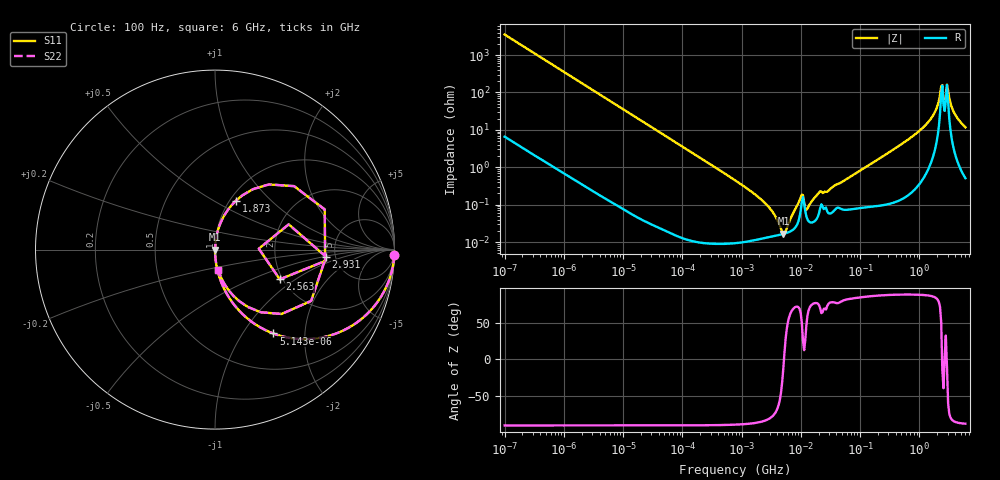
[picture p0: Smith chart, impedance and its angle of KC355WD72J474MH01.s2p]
!Murata Part Number: KC355WD72J474MH01
!These Parameters are Measured in Series Mode Connection
!Data Generated on Mar 13, 2026
!  o--ll--o
!Port1  Port2
!  o------o
!Operation Temp=25[degC], DC Bias Voltage=0[V]
!Freq. Start=100[Hz] Stop=6[GHz] 401[Steps]
# Hz S RI R 50
!Freq.(Hz) S11(Real) S11(Imag) S21(Real) S21(Imag) S12(Real) S12(Imag) S22(Real) S22(Imag)
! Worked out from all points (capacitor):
!   401 points, 100 Hz to 6 GHz, reference 50 ohm
!   read as one part in series: C = 449 nF near 109 Hz
!   lowest |Z| = 16.8 mohm at 5.079 MHz (marker M1)
!   series resonance near 5.199 MHz, so ESL is about 2.1 nH
!   S11 on the Smith chart (normalised r, x): 100 Hz: 1, -71; 5.143 kHz: 1.00, -1.39; 1.873 GHz: 1.07, +0.64; 2.563 GHz: 1.93, -0.76; 2.931 GHz: 4.19, -0.55; 6 GHz: 1.01, -0.23
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100  0.9992 -0.0282  0.000847 0.0282  0.000847 0.0282  0.9992 -0.0282
750  0.957 -0.2019  0.043 0.2019  0.043 0.2019  0.957 -0.2019
2008  0.758 -0.4273  0.242 0.4273  0.242 0.4273  0.758 -0.4273
5143  0.3246 -0.4672  0.6754 0.4672  0.6754 0.4672  0.3246 -0.4672
12041  0.0811 -0.272  0.9189 0.272  0.9189 0.272  0.0811 -0.272
40335  0.00801 -0.0878  0.992 0.0878  0.992 0.0878  0.00801 -0.0878
774597  0.000113 -0.0045  0.9999 0.0045  0.9999 0.0045  0.000113 -0.0045
2713602  0.000133 -0.000948  0.9999 0.000948  0.9999 0.000948  0.000133 -0.000948
5079039  0.000165 -3.23e-05  0.9998 3.23e-05  0.9998 3.23e-05  0.000165 -3.23e-05
9941735  0.000696 0.00138  0.9993 -0.00138  0.9993 -0.00138  0.000696 0.00138
1.300572e7  0.000397 0.0007  0.9996 -0.0007  0.9996 -0.0007  0.000397 0.0007
1.555665e7  0.000336 0.00123  0.9997 -0.00123  0.9997 -0.00123  0.000336 0.00123
2.035112e7  0.000605 0.00205  0.9994 -0.00205  0.9994 -0.00205  0.000605 0.00205
3.124326e8  0.00169 0.0252  0.9983 -0.0252  0.9983 -0.0252  0.00169 0.0252
1.046602e9  0.0136 0.0979  0.9864 -0.0979  0.9864 -0.0979  0.0136 0.0979
1.873145e9  0.1164 0.2723  0.8836 -0.2723  0.8836 -0.2723  0.1164 0.2723
2.240541e9  0.4405 0.3536  0.5595 -0.3536  0.5595 -0.3536  0.4405 0.3536
2.562649e9  0.3609 -0.1657  0.6391 0.1657  0.6391 0.1657  0.3609 -0.1657
2.931063e9  0.6189 -0.0403  0.3811 0.0403  0.3811 0.0403  0.6189 -0.0403
3.352442e9  0.2549 -0.3491  0.7451 0.3491  0.7451 0.3491  0.2549 -0.3491
4.009986e9  0.0814 -0.2331  0.9186 0.2331  0.9186 0.2331  0.0814 -0.2331
6e9  0.0184 -0.1143  0.9816 0.1143  0.9816 0.1143  0.0184 -0.1143
